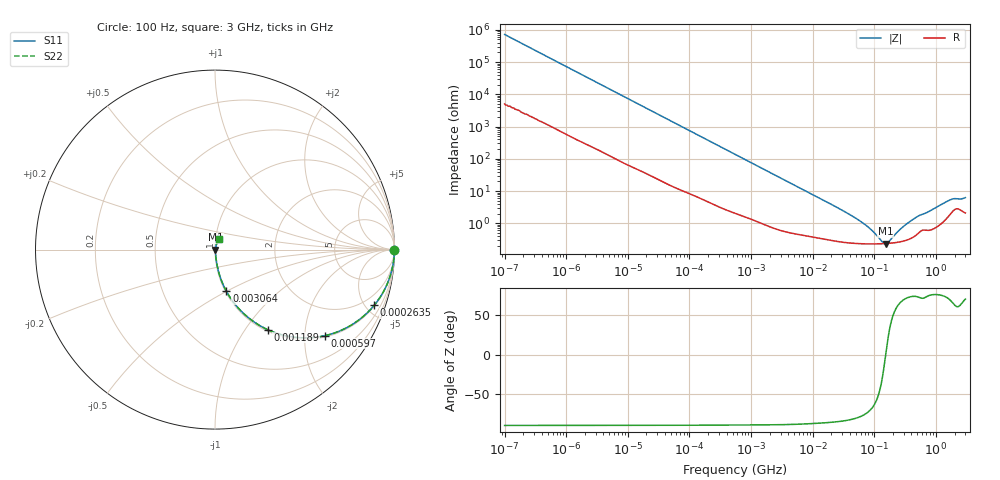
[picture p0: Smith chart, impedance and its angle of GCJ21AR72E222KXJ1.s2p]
!Murata Part Number: GCJ21AR72E222KXJ1
!These Parameters are Measured in Series Mode Connection
!Data Generated on Mar 13, 2026
!  o--ll--o
!Port1  Port2
!  o------o
!Operation Temp=25[degC], DC Bias Voltage=0[V]
!Freq. Start=100[Hz] Stop=3[GHz] 401[Steps]
# Hz S RI R 50
!Freq.(Hz) S11(Real) S11(Imag) S21(Real) S21(Imag) S12(Real) S12(Imag) S22(Real) S22(Imag)
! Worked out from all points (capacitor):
!   401 points, 100 Hz to 3 GHz, reference 50 ohm
!   read as one part in series: C = 2.22 nF near 109 Hz
!   lowest |Z| = 236 mohm at 153.9 MHz (marker M1)
!   series resonance near 152.6 MHz, so ESL is about 490 pH
!   S11 on the Smith chart (normalised r, x): 100 Hz: open; 263.5 kHz: 1.07, -5.68; 597 kHz: 1.04, -2.52; 1.189 MHz: 1.02, -1.28; 3.064 MHz: 1.01, -0.50; 3 GHz: 1.04, +0.12
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100  1 -0.00014  1e-06 0.00014  1e-06 0.00014  1 -0.00014
1788  1 -0.00246  2.6e-05 0.00246  2.6e-05 0.00246  1 -0.00246
31977  0.9977 -0.0432  0.00229 0.0432  0.00229 0.0432  0.9977 -0.0432
102221  0.98 -0.1346  0.02 0.1346  0.02 0.1346  0.98 -0.1346
263501  0.8867 -0.3107  0.1133 0.3107  0.1133 0.3107  0.8867 -0.3107
371814  0.7996 -0.3936  0.2004 0.3936  0.2004 0.3936  0.7996 -0.3936
547723  0.6515 -0.4691  0.3485 0.4691  0.3485 0.4691  0.6515 -0.4691
596961  0.6124 -0.4796  0.3876 0.4796  0.3876 0.4796  0.6124 -0.4796
842342  0.4467 -0.4888  0.5533 0.4888  0.5533 0.4888  0.4467 -0.4888
1188587  0.2927 -0.4459  0.7073 0.4459  0.7073 0.4459  0.2927 -0.4459
1827928  0.1528 -0.3499  0.8472 0.3499  0.8472 0.3499  0.1528 -0.3499
3063887  0.0635 -0.2322  0.9365 0.2322  0.9365 0.2322  0.0635 -0.2322
9794414  0.00988 -0.0777  0.9901 0.0777  0.9901 0.0777  0.00988 -0.0777
5.478864e7  0.0025 -0.0125  0.9975 0.0125  0.9975 0.0125  0.0025 -0.0125
8.79653e7  0.00232 -0.006  0.9977 0.006  0.9977 0.006  0.00232 -0.006
1.352818e8  0.00233 -0.00125  0.9977 0.00125  0.9977 0.00125  0.00233 -0.00125
1.539281e8  0.00235 8.87e-05  0.9976 -8.87e-05  0.9976 -8.87e-05  0.00235 8.87e-05
1.751444e8  0.0024 0.00143  0.9976 -0.00143  0.9976 -0.00143  0.0024 0.00143
2.812011e8  0.00278 0.00677  0.9972 -0.00677  0.9972 -0.00677  0.00278 0.00677
4.920662e8  0.00473 0.0151  0.9953 -0.0151  0.9953 -0.0151  0.00473 0.0151
1.71441e9  0.0213 0.0481  0.9787 -0.0481  0.9787 -0.0481  0.0213 0.0481
3e9  0.0238 0.0565  0.9762 -0.0565  0.9762 -0.0565  0.0238 0.0565
